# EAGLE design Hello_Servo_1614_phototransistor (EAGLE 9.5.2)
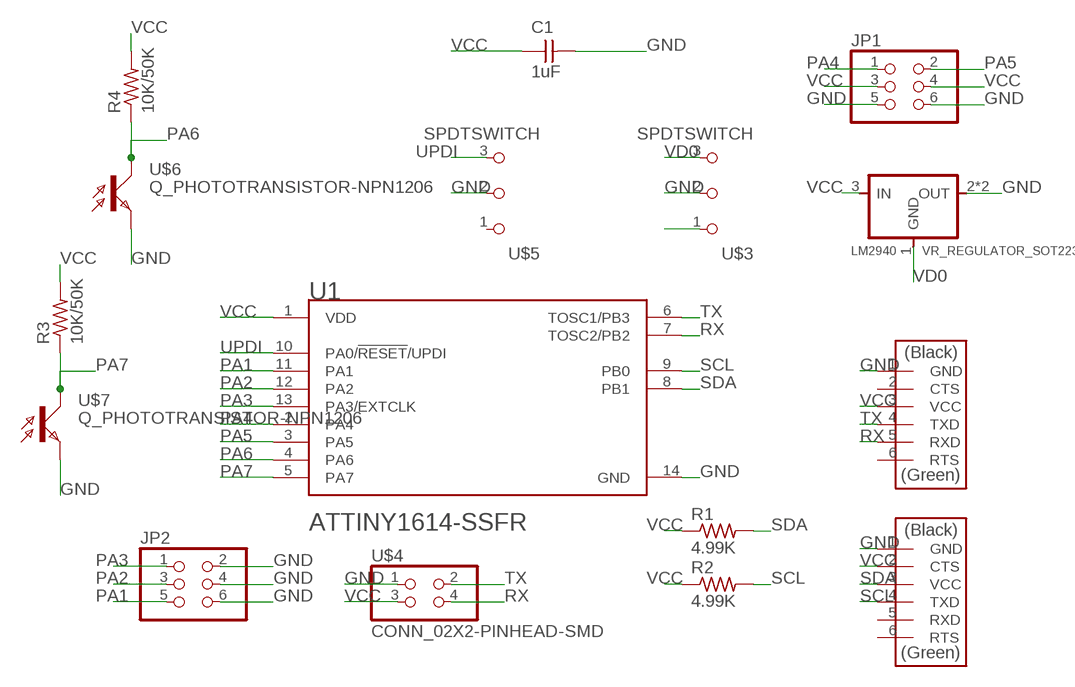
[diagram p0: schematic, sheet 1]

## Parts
C1  1uF  CAP_UNPOLARIZEDFAB  [C1206FAB]
JP1  CONN_03X2-PINHEAD-SMD  [2X03SMD]
JP2  CONN_03X2-PINHEAD-SMD  [2X03SMD]
LM2940  VR_REGULATOR_SOT223  [SOT223]
R1  4.99K  R1206FAB  [R1206FAB]
R2  4.99K  R1206FAB  [R1206FAB]
R3  10K/50K  R1206FAB  [R1206FAB]
R4  10K/50K  R1206FAB  [R1206FAB]
U1  MICROCHIP_ATTINY1614-SSFRMICROCHIP_ATTINY1614-SSFR_0_1  [MICROCHIP_ATTINY1614]
U$1  CONN_06_FTDI-SMD-HEADER  [1X06SMD]
U$2  CONN_06_FTDI-SMD-HEADER  [1X06SMD]
U$3  SPDTSWITCH  [SPDTSWITCH]
U$4  CONN_02X2-PINHEAD-SMD  [2X02SMD]
U$5  SPDTSWITCH  [SPDTSWITCH]
U$6  Q_PHOTOTRANSISTOR-NPN1206  [OP1206]
U$7  Q_PHOTOTRANSISTOR-NPN1206  [OP1206]

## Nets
GND: C1.2 JP1.5 JP1.6 JP2.2 JP2.4 JP2.6 LM2940.2(OUT) LM2940.4(OUT) U1.14(GND) U$1.1(GND) U$2.1(GND) U$3.2 U$4.1 U$5.2 U$6.EMITTER(E) U$7.EMITTER(E)
N$2: U$3.1
PA1: JP2.5 U1.11(PA1)
PA2: JP2.3 U1.12(PA2)
PA3: JP2.1 U1.13(PA3/EXTCLK)
PA4: JP1.1 U1.2(PA4)
PA5: JP1.2 U1.3(PA5)
PA6: R4.1 U1.4(PA6) U$6.COLLECTOR(C)
PA7: R3.1 U1.5(PA7) U$7.COLLECTOR(C)
RX: U1.7(TOSC2/PB2) U$2.5(RXD) U$4.4
SCL: R2.2 U1.9(PB0) U$1.4(TXD)
SDA: R1.2 U1.8(PB1) U$1.3(VCC)
TX: U1.6(TOSC1/PB3) U$2.4(TXD) U$4.2
UPDI: U1.10(PA0/!RESET!/UPDI) U$5.3
VCC [New Class]: C1.1 JP1.3 JP1.4 LM2940.3(IN) R1.1 R2.1 R3.2 R4.2 U1.1(VDD) U$1.2(CTS) U$2.3(VCC) U$4.3
VD0: LM2940.1(GND) U$3.3
Unconnected: U$1.5(RXD) U$1.6(RTS) U$2.2(CTS) U$2.6(RTS) U$5.1

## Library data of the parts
C1 = fab:CAP_UNPOLARIZED
JP1 JP2 = fab:CONN_03X2-PINHEAD-SMD: PIN HEADER
LM2940 = fab:VR_REGULATOR_SOT223
R1-R4 = fab:R: Resistor (US Symbol)
U1 = Microchip - ATTINY1614-SSFR:MICROCHIP_ATTINY1614-SSFR: IC MCU 8BIT 16KB FLASH 14SOIC; AUTOMOTIVE: No; CENTROID_NOT_SPECIFIED: No; CORE_ARCHITECTURE: AVR; DATASHEET: http://ww1.microchip.com/downloads/en/DeviceDoc/ATtiny1614-DataSheet-DS40001995B.pdf; DATA_BUS_WIDTH: 8bits; DEVICE_CLASS_L1: Integrated Circuits (ICs); DEVICE_CLASS_L2: Embedded Processors and Controllers; DEVICE_CLASS_L3: Microcontrollers; DIGIKEY_DESCRIPTION: IC MCU 8BIT 16KB FLASH 14SOIC; DIGIKEY_PART_NUMBER: ATTINY1614-SSFRCT-ND; FOOTPRINT_PARAMETERS_1: {"fp_type":"SOIC_narrow","params":{"N":{"nom":14,"long name":"Number of leads","min":null,"max":null,"short name":"N","type":"count"},"A":{"nom":false,"long name":"Height","min":false,"max":1750000,"short name":"A","type":"measurement"},"A1":{"nom":false,"long name":"Package clearance","min":100000,"max":250000,"short name":"A1","type":"measurement"},"A2":{"nom":false,"long name":"Package height","min":1250000,"max":false,"short name":"A2","type":"measurement"},"D":{"nom":8650000,"long name":"Package length","min":8550000,"max":8750000,"short name":"D","type":"measurement"},"E":{"nom":6000000,"long name":"Width w/ leads","min":5800000,"max":6200000,"short name":"E","type":"measurement"},"E1":{"nom":3900000,"long name":"Package width","min":3800000,"max":4000000,"short name":"E1","type":"measurement"},"B":{"nom":false,"long name":"Lead width","min":310000,"max":510000,"short name":"B","type":"measurement"},"C":{"nom":false,"long name":"Lead thickness","min":100000,"max":250000,"short name":"C","type":"measurement"},"e":{"nom":1270000,"long name":"Lead pitch","min":null,"max":null,"short name":"e","type":"measurement"},"L":{"nom":false,"long name":"Lead foot length","min":400000,"max":1270000,"short name":"L","type":"measurement"},"PHI":{"nom":false,"long name":"Lead foot angle","min":0,"max":8000000,"short name":"PHI","type":"measurement"},"HT":{"default":"No","long name":"Thermal pad","type":"multichoiceparent","short name":"HT","children":[]},"offset x":{"nom":0,"long name":"X Center offset","min":null,"max":null,"short name":"offset x","type":"measurement"},"offset y":{"nom":0,"long name":"Y Center offset","min":null,"max":null,"short name":"offset y","type":"measurement"},"LS":{"default":"Rounded rectangle","long name":"Land shape","type":"multichoice","short name":"LS"},"LS1":{"default":"Rectangle","long name":"Land shape (Pin 1)","type":"multichoice","short name":"LS1"},"solder toe":{"nom":550000,"long name":"Solder fillet (toe)","min":null,"max":null,"short name":"solder toe","type":"fixedmeasurement"},"solder heel":{"nom":450000,"long name":"Solder fillet (heel)","min":null,"max":null,"short name":"solder heel","type":"fixedmeasurement"},"solder side":{"nom":50000,"long name":"Solder fillet (side)","min":null,"max":null,"short name":"solder side","type":"fixedmeasurement"},"courtyard":{"nom":500000,"long name":"Courtyard","min":null,"max":null,"short name":"courtyard","type":"fixedmeasurement"},"SF":{"default":"A","long name":"Packing level","type":"multichoiceparent","short name":"SF","help":"http://support.upverter.com/customer/portal/articles/978783-what-is-a-footprint-packing-level","children":["solder toe","solder heel","solder side","courtyard"]}}}; FOOTPRINT_PARAMETERS_2: {"fp_type":"SOIC_narrow","params":{"N":{"nom":14,"long name":"Number of leads","min":null,"max":null,"short name":"N","type":"count"},"A":{"nom":false,"long name":"Height","min":false,"max":1750000,"short name":"A","type":"measurement"},"A1":{"nom":false,"long name":"Package clearance","min":100000,"max":250000,"short name":"A1","type":"measurement"},"A2":{"nom":false,"long name":"Package height","min":1250000,"max":false,"short name":"A2","type":"measurement"},"D":{"nom":8650000,"long name":"Package length","min":8550000,"max":8750000,"short name":"D","type":"measurement"},"E":{"nom":6000000,"long name":"Width w/ leads","min":5800000,"max":6200000,"short name":"E","type":"measurement"},"E1":{"nom":3900000,"long name":"Package width","min":3800000,"max":4000000,"short name":"E1","type":"measurement"},"B":{"nom":false,"long name":"Lead width","min":310000,"max":510000,"short name":"B","type":"measurement"},"C":{"nom":false,"long name":"Lead thickness","min":100000,"max":250000,"short name":"C","type":"measurement"},"e":{"nom":1270000,"long name":"Lead pitch","min":null,"max":null,"short name":"e","type":"measurement"},"L":{"nom":false,"long name":"Lead foot length","min":400000,"max":1270000,"short name":"L","type":"measurement"},"PHI":{"nom":false,"long name":"Lead foot angle","min":0,"max":8000000,"short name":"PHI","type":"measurement"},"HT":{"default":"No","long name":"Thermal pad","type":"multichoiceparent","short name":"HT","children":[]},"offset x":{"nom":0,"long name":"X Center offset","min":null,"max":null,"short name":"offset x","type":"measurement"},"offset y":{"nom":0,"long name":"Y Center offset","min":null,"max":null,"short name":"offset y","type":"measurement"},"LS":{"default":"Rounded rectangle","long name":"Land shape","type":"multichoice","short name":"LS"},"LS1":{"default":"Rectangle","long name":"Land shape (Pin 1)","type":"multichoice","short name":"LS1"},"solder toe":{"nom":350000,"long name":"Solder fillet (toe)","min":null,"max":null,"short name":"solder toe","type":"fixedmeasurement"},"solder heel":{"nom":350000,"long name":"Solder fillet (heel)","min":null,"max":null,"short name":"solder heel","type":"fixedmeasurement"},"solder side":{"nom":30000,"long name":"Solder fillet (side)","min":null,"max":null,"short name":"solder side","type":"fixedmeasurement"},"courtyard":{"nom":250000,"long name":"Courtyard","min":null,"max":null,"short name":"courtyard","type":"fixedmeasurement"},"SF":{"default":"B","long name":"Packing level","type":"multichoiceparent","short name":"SF","help":"http://support.upverter.com/customer/portal/articles/978783-what-is-a-footprint-packing-level","children":["solder toe","solder heel","solder side","courtyard"]}}}; FOOTPRINT_PARAMETERS_3: {"fp_type":"SOIC_narrow","params":{"N":{"nom":14,"long name":"Number of leads","min":null,"max":null,"short name":"N","type":"count"},"A":{"nom":false,"long name":"Height","min":false,"max":1750000,"short name":"A","type":"measurement"},"A1":{"nom":false,"long name":"Package clearance","min":100000,"max":250000,"short name":"A1","type":"measurement"},"A2":{"nom":false,"long name":"Package height","min":1250000,"max":false,"short name":"A2","type":"measurement"},"D":{"nom":8650000,"long name":"Package length","min":8550000,"max":8750000,"short name":"D","type":"measurement"},"E":{"nom":6000000,"long name":"Width w/ leads","min":5800000,"max":6200000,"short name":"E","type":"measurement"},"E1":{"nom":3900000,"long name":"Package width","min":3800000,"max":4000000,"short name":"E1","type":"measurement"},"B":{"nom":false,"long name":"Lead width","min":310000,"max":510000,"short name":"B","type":"measurement"},"C":{"nom":false,"long name":"Lead thickness","min":100000,"max":250000,"short name":"C","type":"measurement"},"e":{"nom":1270000,"long name":"Lead pitch","min":null,"max":null,"short name":"e","type":"measurement"},"L":{"nom":false,"long name":"Lead foot length","min":400000,"max":1270000,"short name":"L","type":"measurement"},"PHI":{"nom":false,"long name":"Lead foot angle","min":0,"max":8000000,"short name":"PHI","type":"measurement"},"HT":{"default":"No","long name":"Thermal pad","type":"multichoiceparent","short name":"HT","children":[]},"offset x":{"nom":0,"long name":"X Center offset","min":null,"max":null,"short name":"offset x","type":"measurement"},"offset y":{"nom":0,"long name":"Y Center offset","min":null,"max":null,"short name":"offset y","type":"measurement"},"LS":{"default":"Rounded rectangle","long name":"Land shape","type":"multichoice","short name":"LS"},"LS1":{"default":"Rectangle","long name":"Land shape (Pin 1)","type":"multichoice","short name":"LS1"},"solder toe":{"nom":150000,"long name":"Solder fillet (toe)","min":null,"max":null,"short name":"solder toe","type":"fixedmeasurement"},"solder heel":{"nom":250000,"long name":"Solder fillet (heel)","min":null,"max":null,"short name":"solder heel","type":"fixedmeasurement"},"solder side":{"nom":10000,"long name":"Solder fillet (side)","min":null,"max":null,"short name":"solder side","type":"fixedmeasurement"},"courtyard":{"nom":100000,"long name":"Courtyard","min":null,"max":null,"short name":"courtyard","type":"fixedmeasurement"},"SF":{"default":"C","long name":"Packing level","type":"multichoiceparent","short name":"SF","help":"http://support.upverter.com/customer/portal/articles/978783-what-is-a-footprint-packing-level","children":["solder toe","solder heel","solder side","courtyard"]}}}; FOOTPRINT_VARIANT_NAME_0: Recommended_Land_Pattern; FOOTPRINT_VARIANT_NAME_1: IPC_A; FOOTPRINT_VARIANT_NAME_2: IPC_B; FOOTPRINT_VARIANT_NAME_3: IPC_C; FREQUENCY: 16MHz; HEIGHT: 1.75mm; INTERFACE: I2C,SPI,UART,USART,2-Wire,LIN,IrDA; IPC_LAND_PATTERN_NAME: SOIC127P600X175-14; LEAD_FREE: Yes; MAX_SUPPLY_VOLTAGE: 5.5V; MEMORY_SIZE: 16KBytes; MEMORY_TYPE: FLASH; MF: Microchip; MFG_PACKAGE_IDENT: C04-065-D3X; MFG_PACKAGE_IDENT_DATE: 0; MFG_PACKAGE_IDENT_REV: D; MIN_SUPPLY_VOLTAGE: 1.8V; MOUSER_DESCRIPTION: 8-Bit AVR Microcontroller 16Kbyte Flash 2Kbyte SRAM 14-Pin SOIC T/R; MOUSER_PART_NUMBER: 556-ATTINY1614SSFR; MPN: ATTINY1614-SSFR; NOMINAL_SUPPLY_CURRENT: 2.6-10200uA; NUMBER_OF_A/D_CONVERTERS: 2; NUMBER_OF_ADC_CHANNELS: 14; NUMBER_OF_CORES: 1; NUMBER_OF_I/OS: 12; NUMBER_OF_I2C_CHANNELS: 1; NUMBER_OF_PWM_CHANNELS: 1; NUMBER_OF_SPI_CHANNELS: 1; NUMBER_OF_TIMERS/COUNTERS: 5; NUMBER_OF_UART_CHANNELS: 1; PACKAGE: SOIC14; PREFIX: U; RAM_SIZE: 2KBytes; ROHS: Yes; STANDOFF_HEIGHT: 0.1mm; TEMPERATURE_RANGE_HIGH: +125°C; TEMPERATURE_RANGE_LOW: -40°C; VERIFICATION_VERSION: 0.0.0.3
U$1 U$2 = fab:CONN_06_FTDI-SMD-HEADER
U$3 U$5 = fab:SPDTSWITCH
U$4 = fab:CONN_02X2-PINHEAD-SMD
U$6 U$7 = fab:Q_PHOTOTRANSISTOR-NPN

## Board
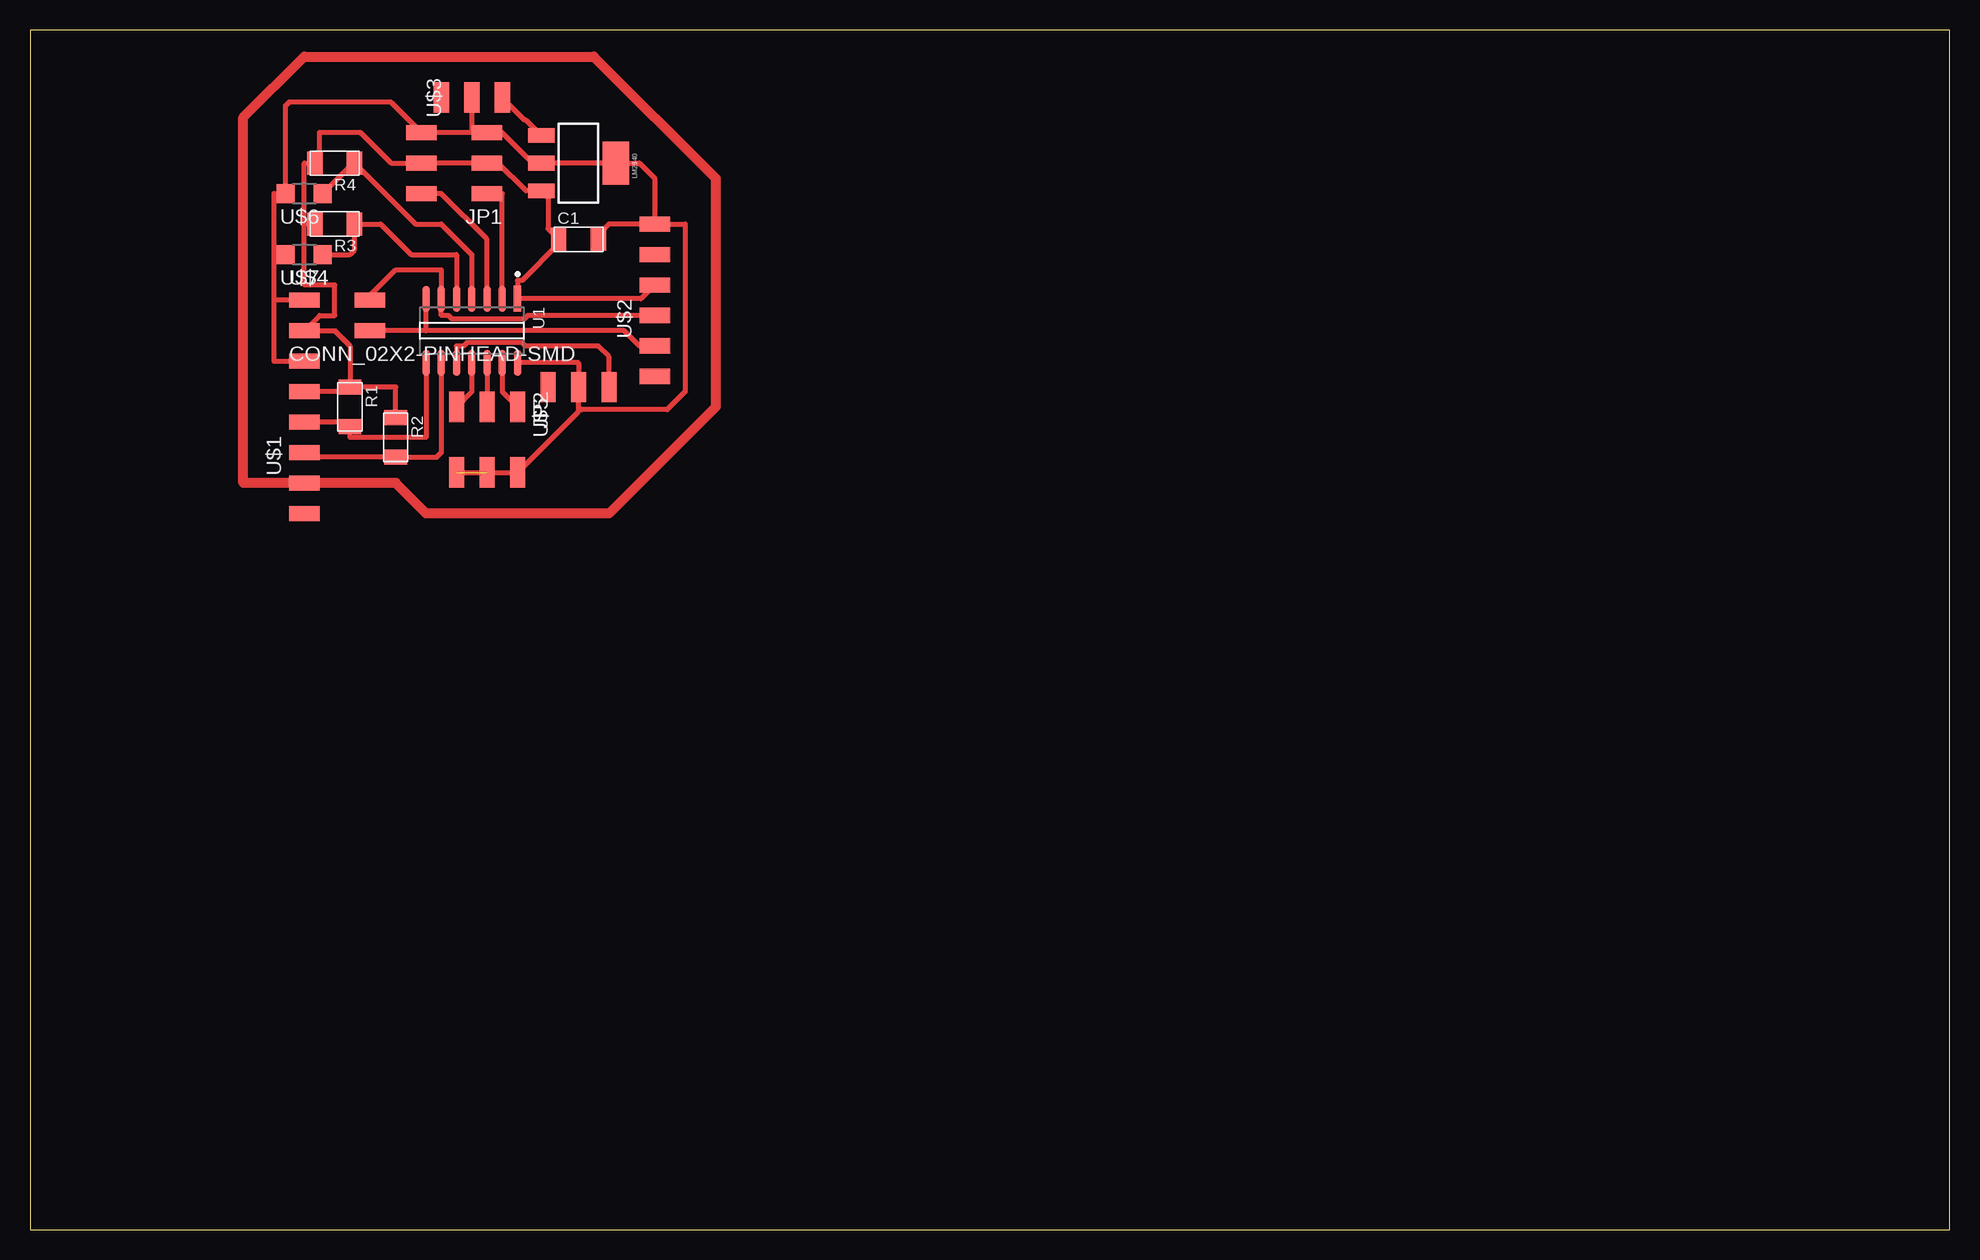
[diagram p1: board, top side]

Size 160 x 100 mm. Coordinates in mm from the lower left corner, seen from the top.
Outline: 0,0 160,0 160,100 0,100 0,0
Copper layers (1*16): Top 0.035mm / dielectric 1.5mm / Bottom 0.035mm
Design rules "default *": minimum track width 16mil, minimum drill 0.35mm, track to track 16mil, track to pad 16mil, pad to pad 16mil, via to via 16mil, smd to smd 6mil, copper to edge 40mil, drill to drill 6mil, minimum pad ring 10mil, minimum via ring 8mil, stop-mask expansion 4mil, vias tented up to drill 0mil, thermal gap 10mil

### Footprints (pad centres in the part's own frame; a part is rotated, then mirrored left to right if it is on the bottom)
C1206FAB = smd 1.27 x 1.905: 1 -1.651,0; 2 1.651,0
2X03SMD = smd 2.54 x 1.27: 1 -2.54,2.54; 2 2.92,2.54; 3 -2.54,0; 4 2.92,0; 5 -2.54,-2.54; 6 2.92,-2.54
SOT223 = smd 1.219 x 2.235: 1 -2.311,-3.099; 2 0,-3.099; 3 2.311,-3.099 | smd 3.6 x 2.2: 4 0,3.099
R1206FAB = smd 1.27 x 1.905: 1 -1.651,0; 2 1.651,0
MICROCHIP_ATTINY1614 = smd 2.169 x 0.622: 1 -2.67,3.81; 2 -2.67,2.54; 3 -2.67,1.27; 4 -2.67,0; 5 -2.67,-1.27; 6 -2.67,-2.54; 7 -2.67,-3.81; 8 2.67,-3.81; 9 2.67,-2.54; 10 2.67,-1.27; 11 2.67,0; 12 2.67,1.27; 13 2.67,2.54; 14 2.67,3.81
1X06SMD = smd 2.54 x 1.27: 1 0,6.35; 2 0,3.81; 3 0,1.27; 4 0,-1.27; 5 0,-3.81; 6 0,-6.35
SPDTSWITCH = smd 2.54 x 1.27: 1 0.38,2.54; 2 0.38,0; 3 0.38,-2.54
2X02SMD = smd 2.54 x 1.27: 1 -2.54,1.27; 2 2.92,1.27; 3 -2.54,-1.27; 4 2.92,-1.27
OP1206 = smd 1.5 x 1.6: COLLECTOR -1.55,0; EMITTER 1.55,0

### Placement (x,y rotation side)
C1  45.72,82.55 0 top
JP1  35.56,88.9 180 top
JP2  38.1,66.04 270 top
LM2940  45.72,88.9 270 top
R1  26.67,68.58 270 top
R2  30.48,66.04 270 top
R3  25.4,83.82 180 top
R4  25.4,88.9 180 top
U1  36.83,74.93 270 top
U$1  22.86,66.04 0 top
U$2  52.07,77.47 0 top
U$3  36.83,93.98 90 top
U$4  25.4,76.2 0 top
U$5  45.72,69.85 90 top
U$6  22.86,86.36 180 top
U$7  22.86,81.28 180 top

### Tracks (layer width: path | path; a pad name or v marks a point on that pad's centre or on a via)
GND  (1 unrouted)
  Top 0.406: U1.14 45.72,72.26 U$5.2 | U$3.2 36.83,91.44 JP1.5 | U$2.1 52.07,87.63 50.8,88.9 LM2940.4 LM2940.2 41.91,88.9 39.37,91.44 JP1.5 | JP1.5 JP1.6 | U$2.1 54.61,83.82 54.61,69.85 53.11,68.35 45.95,68.35 45.72,68.58 U$5.2 | 31.75,91.44 JP1.6 | U$4.1 20.32,77.47 | 20.32,77.47 20.32,72.39 U$1.1 | 20.32,81.28 20.32,86.36 U$6.EMITTER 21.31,93.7 21.59,93.98 30.1,93.98 JP1.6 | 20.32,81.28 20.32,77.47 | JP2.6 JP2.2 45.72,68.2 U$5.2 | U$2.1 48.26,83.82 47.37,82.93 C1.2 | U$7.EMITTER 20.32,81.28
N$1
  Top 0.813: 22.86,97.79 46.99,97.79 57.15,87.63 57.15,68.58 48.26,59.69 33.02,59.69 30.48,62.23 17.78,62.23 17.78,92.71 22.86,97.79
PA1
  Top 0.406: U1.11 36.83,69.85 JP2.5
PA2
  Top 0.406: U1.12 JP2.3
PA3
  Top 0.406: U1.13 39.37,69.85 JP2.1
PA4
  Top 0.406: JP1.1 39.37,86.36 U1.2
PA5
  Top 0.406: U1.3 38.1,82.55 34.29,86.36 JP1.2
PA6
  Top 0.406: U1.4 36.83,81.28 34.29,83.82 32.13,83.82 R4.1 26.95,88.9 U$6.COLLECTOR
PA7
  Top 0.406: U$7.COLLECTOR 26.67,81.28 27.05,81.66 R3.1 29.21,83.82 31.75,81.28 35.56,81.28 U1.5
RX
  Top 0.406: U$2.5 50.8,73.66 49.53,74.93 33.02,74.93 | 33.02,74.93 U1.7 | 33.02,74.93 U$4.4
SCL
  Top 0.406: U1.9 34.29,64.77 33.91,64.39 R2.2 23.24,64.39 U$1.4
SDA
  Top 0.406: U1.8 33.02,66.04 26.67,66.04 R1.2 26.29,67.31 U$1.3
TX
  Top 0.406: U$2.4 41.5,76.2 41.2,75.91 35.18,75.91 34.88,76.2 34.29,76.2 34.29,77.47 U1.6 34.29,80.01 30.48,80.01 28.32,77.85 U$4.2
UPDI
  Top 0.406: U$5.3 48.26,72.77 47.37,73.66 41.32,73.66 41.02,73.95 36.45,73.95 36.15,73.66 35.56,73.66 U1.10
VCC
  Top 0.406: U$2.3 50.93,77.6 U1.1 40.64,79.12 41.02,79.12 44.07,82.17 C1.1 43.18,83.44 43.18,86.03 LM2940.3 41.35,86.59 39.04,88.9 JP1.3 JP1.4 | R2.1 30.48,70.23 R1.1 | R1.1 26.29,69.85 U$1.2 | R1.1 26.67,73.66 25.4,74.93 U$4.3 24.13,76.2 25.4,76.2 25.4,78.74 22.86,78.74 22.86,83.82 | 31.75,88.9 JP1.4 | JP1.4 30.1,88.9 27.56,91.44 24.13,91.44 24.13,89.28 R4.2 22.86,88.9 22.86,83.82 | R3.2 22.86,83.82
VD0
  Top 0.406: U$3.3 41.25,92.48 41.35,92.48 LM2940.1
